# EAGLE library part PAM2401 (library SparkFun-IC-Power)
PAM2401 - Boost PMIC Specifications: Up to 1A output current 0.9V to 4.75V Input Range 2.5V to 5.0V Adjustable Output Voltage Datasheet (Diodes inc.)
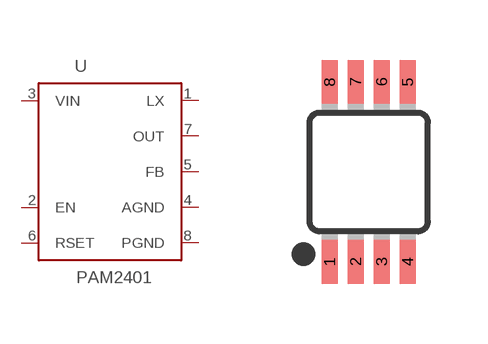
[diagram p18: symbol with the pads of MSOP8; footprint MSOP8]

Designator prefix -

## PAM2401 (PROD_ID: IC-13769; VALUE: PAM2401)  [MSOP8]
1  LX
2  EN
3  VIN
4  AGND
5  FB
6  RSET
7  OUT
8  PGND

## Footprint MSOP8 (pad centres in mm)
8M, 8-Lead, 0.118" Wide, Miniature Small Outline Package MSOP 8M-Package doc1097.pdf
smd 0.4 x 1.1: 1 -0.975,-2.25; 2 -0.325,-2.25; 3 0.325,-2.25; 4 0.975,-2.25; 5 0.975,2.25; 6 0.325,2.25; 7 -0.325,2.25; 8 -0.975,2.25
